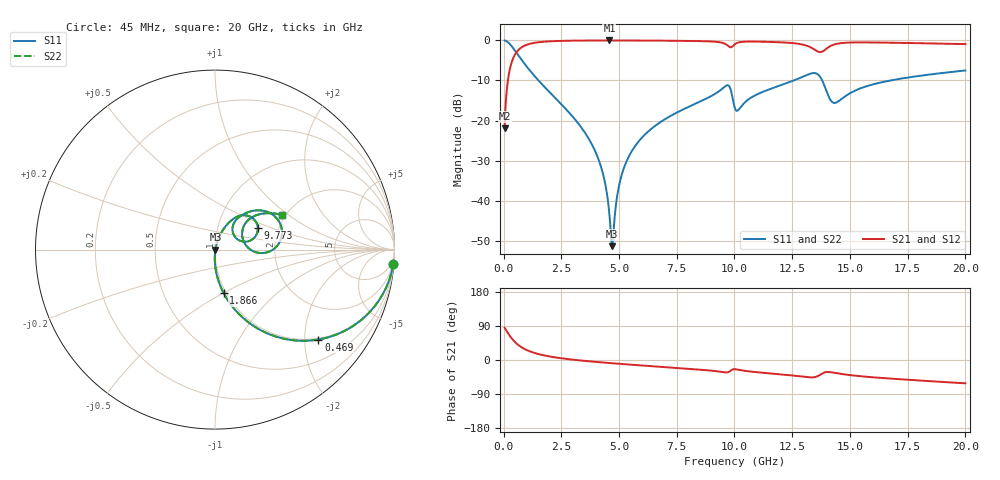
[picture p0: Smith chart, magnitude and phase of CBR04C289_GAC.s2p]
! S-parameter model data by Modelithics Inc.  support@modelithics.com 813-866-6335  Tampa FL USA
! S-Parameter data specifications:
! Substrate: 20-mil Rogers 4350B, substrate thickness, H=0.508mm, Dielectric constant, Er=3.75
! PCB Mounting Pad Footprint: Pad width, PadW=0.52mm , Pad length, PadL=0.52mm , Pad gap, PadG (edge-to-edge)=0.28mm , Reference planes=1.32mm apart
#  GHz  S  MA  R 50
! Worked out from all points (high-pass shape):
!   801 points, 45 MHz to 20 GHz, reference 50 ohm
!   highest |S21| = -0.02 dB at 4.585 GHz (marker M1); lowest = -21.9 dB at 45 MHz (marker M2)
!   |S21| within 3 dB of the highest: 552.5 MHz to end of sweep
!   lowest |S11| = -51.4 dB at 4.709 GHz (marker M3), VSWR 1.01, Z = 50.3 + j0.000814 ohm
!   |S11| at or under -10 dB: 1.511 GHz to 12.57 GHz (11.06 GHz wide, 157 % of centre); 13.8 GHz to 16.77 GHz (2.969 GHz wide, 19.4 % of centre)
!   |S22| runs from -51.4 to 0.0 dB; largest |S21 - S12| = 0
!   S11 on the Smith chart (normalised r, x): 45 MHz: 1, -24; 469 MHz: 0.97, -2.33; 1.866 GHz: 0.97, -0.50; 9.773 GHz: 1.56, +0.41; 20 GHz: 1.92, +0.90
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0.045  0.9967 -4.7  0.0801 85.2  0.0801 85.2  0.9967 -4.7
0.24455  0.9159 -24.1  0.4004 65.9  0.4004 65.9  0.9159 -24.1
0.469044  0.7636 -41.0  0.6448 48.9  0.6448 48.9  0.7636 -41.0
1.017806  0.4649 -64.0  0.8841 25.8  0.8841 25.8  0.4649 -64.0
1.865894  0.246 -78.8  0.9675 10.8  0.9675 10.8  0.246 -78.8
3.387462  0.08031 -90.0  0.9944 -1.6  0.9944 -1.6  0.08031 -90.0
4.210606  0.02698 -90.8  0.997 -6.2  0.997 -6.2  0.02698 -90.8
4.4351  0.01446 -87.0  0.9972 -7.3  0.9972 -7.3  0.01446 -87.0
4.584763  0.006684 -74.8  0.9972 -8.0  0.9972 -8.0  0.006684 -74.8
4.709481  0.002706 0.2  0.9972 -8.6  0.9972 -8.6  0.002706 0.2
4.983862  0.01459 69.1  0.997 -9.9  0.997 -9.9  0.01459 69.1
5.308131  0.03015 73.1  0.9965 -11.4  0.9965 -11.4  0.03015 73.1
6.704981  0.09178 70.3  0.9921 -17.5  0.9921 -17.5  0.09178 70.3
9.42385  0.2433 51.7  0.94 -31.2  0.94 -31.2  0.2433 51.7
9.773062  0.2676 26.8  0.831 -30.9  0.831 -30.9  0.2676 26.8
10.0225  0.1415 22.3  0.8971 -24.2  0.8971 -24.2  0.1415 22.3
11.69373  0.256 50.9  0.9533 -36.2  0.9533 -36.2  0.256 50.9
13.36496  0.3888 24.5  0.7993 -45.9  0.7993 -45.9  0.3888 24.5
13.86384  0.2863 -3.3  0.742 -33.6  0.742 -33.6  0.2863 -3.3
14.33777  0.1656 19.5  0.8918 -33.8  0.8918 -33.8  0.1656 19.5
16.68248  0.3129 38.8  0.9356 -48.7  0.9356 -48.7  0.3129 38.8
20  0.4208 27.2  0.8977 -61.6  0.8977 -61.6  0.4208 27.2
